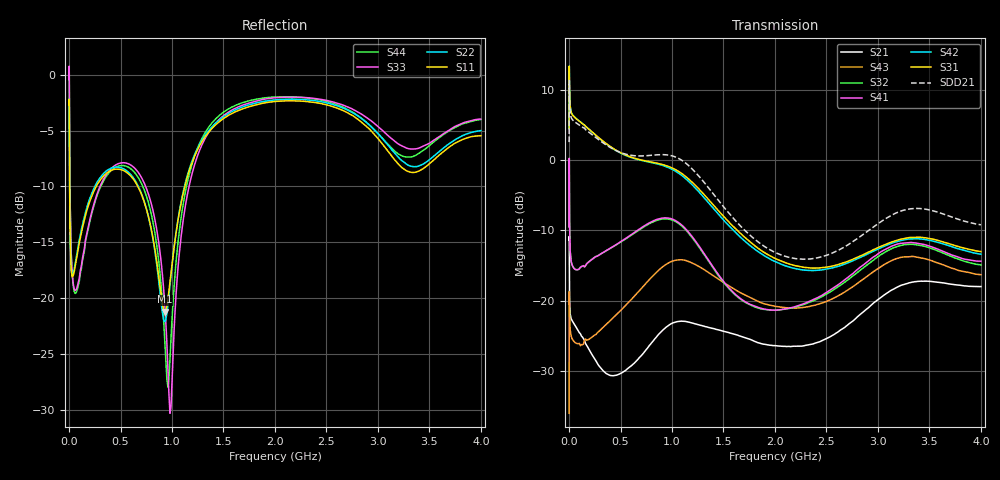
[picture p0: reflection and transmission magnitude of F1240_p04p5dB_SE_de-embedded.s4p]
! Integrated Device Technology
! Corporate Headquarters
! 6024 Silver Creek Valley Road
! San Jose, CA 95138  USA
! Phone:  1-408-284-8200
! Toll Free:  1-800-223-1366
! Webpage:  http://www.idt.com/
! Timing and RF Division
! 515 Groton Road, Suite 102
! Westford, MA 01886-6024
! Device:  F1240
! Description: Dual Intermediate Frequency Digital Variable Gain Amplifier
! Frequency:  10.0 -  500.00 MHz
! Package:  5x5 mm QFN Plastic Package: 32 pin
! Ports:  8 RF, 20 DC
!  Pin  1  = GA3 / Data  Pin 17  = RF OUT_B+
!  Pin  2  = GA4 / CLK  Pin 18  = RF OUT_B-
!  Pin  3  = GA5  Pin 19  = STBY_B
!  Pin  4  = VMODE  Pin 20  = Ground
!  Pin  5  = No Connect  Pin 21  = Ground
!  Pin  6  = GB5  Pin 22  = STB_A
!  Pin  7  = GB4  Pin 23  = RF OUT_A-  = Port 4
!  Pin  8  = GB3  Pin 24  = RF OUT_A+  = Port 3
!  Pin  9  = GB2  Pin 25  = GA0
!  Pin 10  = GB1  Pin 26  = ISET_A
!  Pin 11  = RF IN_B+  Pin 27  = VCC
!  Pin 12  = RF IN_B-  Pin 28  = Ground
!  Pin 13  = Ground  Pin 29  = RF IN_A-  = Port 2
!  Pin 14  = VCC  Pin 30  = RF IN_A+  = Port 1
!  Pin 15  = ISET_B  Pin 31  = GA1
!  Pin 16  = GB0  Pin 32  = GA2 / CSb
! Gain  = +19.5 dB
! State  = 1
! Voltage  = +5.00 V
! Current  = 85.292 mA (one channel only)
! Temperture  =  +25 C
! Test Date  =  2017-10-18
! Board  =  EB4031
! Data:  The device was measured on a custom evaluation board which has
!  individual transmission lines to the RF pins.  Data was collected
!  using a calibrated network analyzer.  The evaluation board was
!  de-embedded using Automatic Fixture Removal.
!  The reference plane is the edge of the package pin.
!  Only Channel A was measured.
!  This data is in single-ended operation.  If your needs are balanced
!  or differential S-parameters then this file needs to be used a
!  linear simulator.
! File Date:  2017-11-10  MJV
! Note:
!  Integrated Device Technology supplies this data as a sample of measured
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# Hz S dB R 100
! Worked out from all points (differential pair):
!   410 points, 500 kHz to 4 GHz, reference 100 ohm
!   strongest paths, dB at 500 kHz, 930 MHz, 1.96 GHz, 2.98 GHz, 4 GHz:
!     S31: 4.5, -0.7, -13.7, -12.6, -13.0
!     S42: 4.5, -0.9, -14.1, -12.8, -13.4
!     S41: -9.5, -8.2, -21.3, -13.6, -14.4
!     S32: -9.5, -8.3, -21.3, -13.9, -14.9
!     S43: -36.0, -14.9, -20.7, -15.6, -16.3
!     S21: -11.4, -23.9, -26.3, -20.1, -18.0
!   taken as a pair (ports 1,2 in; 3,4 out), SDD21 dB: 2.6, 0.8, -12.8, -9.3, -9.2
!   lowest |S11| = -21.2 dB at 930 MHz (marker M1), VSWR 1.19, Z = 85.2 - j6.54 ohm
!   |S11| at or under -10 dB: 5.558 MHz to 263.3 MHz (257.7 MHz wide, 192 % of centre); 667.8 MHz to 1.124 GHz (456.6 MHz wide, 51 % of centre)
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500000  -2.71 -5.5  -11.35 -5.7  -28.49 82.3  -42.45 79.0
        -11.36 -5.7  -2.70 -5.5  -42.44 78.1  -28.49 83.5
        4.50 -105.7  -9.49 -105.4  -0.43 1.2  -36.02 -65.0
        -9.49 -104.3  4.49 -104.5  -35.99 -65.2  -0.44 3.5
2500000  -4.28 -50.5  -14.56 -50.7  -17.37 30.6  -33.39 3.4
         -14.56 -50.8  -4.25 -50.5  -33.34 3.1  -17.38 30.8
         12.90 -177.3  -1.48 159.9  -0.79 -52.6  -18.69 -153.1
         -1.53 160.0  12.89 -177.0  -18.66 -153.1  -0.85 -52.3
3e7  -18.08 -78.8  -22.80 -20.4  -17.74 -8.4  -38.46 -3.6
     -22.81 -20.5  -17.92 -79.6  -38.46 -3.2  -17.72 -8.3
     6.48 161.4  -14.90 139.3  -17.72 -133.5  -25.47 158.0
     -14.93 139.6  6.52 161.4  -25.40 158.0  -17.88 -134.1
1.8e8  -11.92 -123.8  -26.51 -51.7  -19.18 -46.6  -36.41 -4.3
       -26.54 -51.5  -11.66 -125.0  -36.43 -3.5  -19.19 -46.8
       4.55 114.2  -14.60 53.2  -13.89 -126.4  -25.69 100.1
       -14.61 53.3  4.55 113.5  -25.56 99.6  -14.05 -125.6
5.2e8  -8.54 -170.8  -30.42 -65.1  -20.53 -110.2  -31.35 -63.5
       -30.16 -63.8  -8.38 -172.4  -31.46 -61.4  -20.67 -110.6
       0.91 25.1  -11.48 -60.4  -7.88 -167.7  -21.42 9.4
       -11.42 -61.6  0.86 24.0  -21.09 9.0  -8.13 -167.9
9.3e8  -21.20 -154.1  -24.08 -110.2  -19.32 159.6  -28.60 -150.9
       -23.91 -113.7  -22.10 -153.2  -28.68 -144.8  -19.71 158.4
       -0.72 -78.2  -8.35 174.8  -20.65 146.3  -15.32 -92.1
       -8.21 171.6  -0.86 -80.4  -14.94 -93.0  -23.85 163.2
4e9  -5.46 -141.0  -18.02 100.6  -23.70 -56.9  -24.60 -38.9
     -17.97 100.2  -5.00 -139.7  -25.41 -22.5  -25.40 -51.0
     -12.99 26.7  -14.90 -81.8  -3.97 -136.3  -17.40 70.3
     -14.36 -95.7  -13.38 32.7  -16.28 58.5  -4.02 -145.4
